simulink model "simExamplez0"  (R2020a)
settings: Solver=VariableStepAuto  StartTime=0.0  StopTime=tsim  RelTol=1e-3
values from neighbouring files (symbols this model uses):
  df = 0    [runZ0.m]
  td = 1    [runZ0.m]
  tv = 1    [runZ0.m]
  vf = 1    [runZ0.m]    (also in Main.m = v0+dThsp; runTransfOL.m = v00)
undefined symbols (not defined in the file or in its folder): calcu, sysDAE

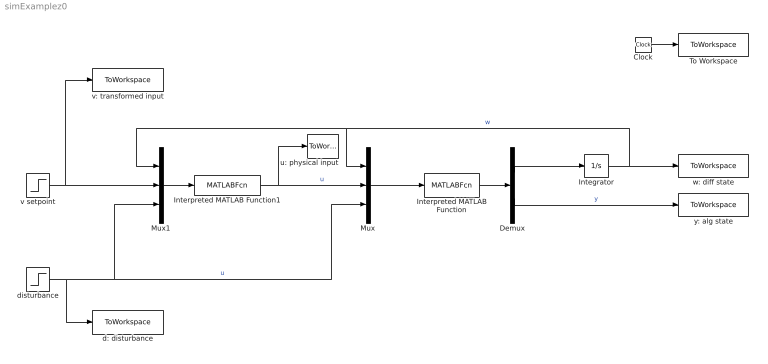
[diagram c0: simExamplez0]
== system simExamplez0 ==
  Clock : Clock
  Demux : Demux  Outputs=2
  Integrator : Integrator
  Interpreted MATLAB Function : MATLABFcn  MATLABFcn=sysDAE(u(1),u(2),u(3))  OutputDimensions=2
  Interpreted MATLAB Function1 : MATLABFcn  MATLABFcn=calcu(u(1),u(2),u(3))  OutputDimensions=1
  Mux : Mux  Inputs=3
  Mux1 : Mux  Inputs=3
  To Workspace : ToWorkspace  VariableName=time  SampleTime=-1
  d: disturbance : ToWorkspace  VariableName=d  SampleTime=-1
  disturbance : Step  Time=td  After=df  SampleTime=0
  u: physical input : ToWorkspace  VariableName=u  SampleTime=-1
  v setpoint : Step  Time=tv  After=vf  SampleTime=0
  v: transformed input : ToWorkspace  VariableName=vs  SampleTime=-1
  w: diff state : ToWorkspace  VariableName=w  SampleTime=-1
  y: alg state : ToWorkspace  VariableName=y  SampleTime=-1
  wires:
  Interpreted MATLAB Function/1 -> Demux/1
  Demux/1 -> Integrator/1
  Integrator/1 -> Mux/1, Mux1/1, w: diff state/1  "w"
  Demux/2 -> y: alg state/1  "y"
  Mux/1 -> Interpreted MATLAB Function/1
  disturbance/1 -> d: disturbance/1, Mux1/3, Mux/3  "u"
  Mux1/1 -> Interpreted MATLAB Function1/1
  v setpoint/1 -> v: transformed input/1, Mux1/2
  Clock/1 -> To Workspace/1
  Interpreted MATLAB Function1/1 -> u: physical input/1, Mux/2  "u"
